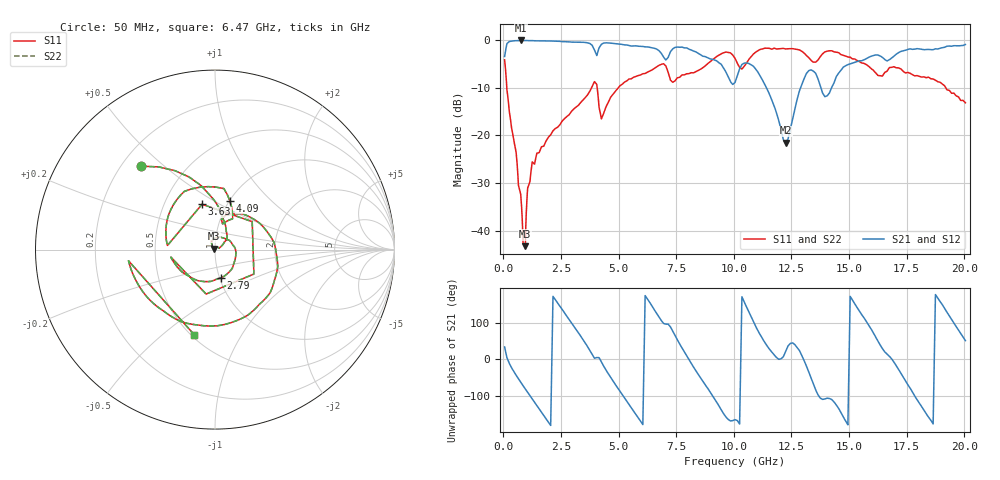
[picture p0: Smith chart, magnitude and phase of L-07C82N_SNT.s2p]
#	mhz	s	ma	r	50
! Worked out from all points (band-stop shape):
!   1001 points, 50 MHz to 20.05 GHz, reference 50 ohm
!   highest |S21| = -0.09 dB at 750 MHz (marker M1); lowest = -21.5 dB at 12.25 GHz (marker M2)
!   |S21| within 3 dB of the highest: 61.95 MHz to 4.037 GHz (3.975 GHz wide, 194 % of centre); 17.02 GHz to end of sweep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
!   lowest |S11| = -43.2 dB at 950 MHz (marker M3), VSWR 1.01, Z = 49.6 + j0.535 ohm
!   |S11| at or under -10 dB: 145.2 MHz to 3.826 GHz (3.681 GHz wide, 185 % of centre); 4.069 GHz to 4.986 GHz (917.5 MHz wide, 20.3 % of centre); 19.2 GHz to end of sweep
!   |S22| runs from -43.2 to -1.7 dB; largest |S21 - S12| = 0
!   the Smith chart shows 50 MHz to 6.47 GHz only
!   S11 on the Smith chart (normalised r, x): 50 MHz: 0.28, +0.42; 2.79 GHz: 1.01, -0.33; 3.63 GHz: 0.77, +0.42; 4.09 GHz: 1.00, +0.60; 6.47 GHz: 0.52, -0.65
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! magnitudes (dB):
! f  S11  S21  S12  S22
! 50 MHz  -4.1  -3.5  -3.5  -4.1
! 750 MHz  -32.4  -0.1  -0.1  -32.4
! 870 MHz  -42.7  -0.1  -0.1  -42.7
! 950 MHz  -43.2  -0.1  -0.1  -43.2
! 1.13 GHz  -29.9  -0.1  -0.1  -29.9
! 1.33 GHz  -25.9  -0.2  -0.2  -25.9
! 2.79 GHz  -15.9  -0.4  -0.4  -15.9
! 3.39 GHz  -12.9  -0.5  -0.5  -12.9
! 3.63 GHz  -11.6  -0.6  -0.6  -11.6
! 4.09 GHz  -10.9  -2.6  -2.6  -10.9
! 4.31 GHz  -15.8  -0.7  -0.7  -15.8
! 6.47 GHz  -6.2  -1.7  -1.7  -6.2
! 6.73 GHz  -5.4  -2.2  -2.2  -5.4
! 7.37 GHz  -8.8  -1.8  -1.8  -8.8
! 10.05 GHz  -3.8  -8.9  -8.9  -3.8
! 10.91 GHz  -2.7  -5.9  -5.9  -2.7
! 12.25 GHz  -1.9  -21.5  -21.5  -1.9
! 13.39 GHz  -4.4  -6.4  -6.4  -4.4
! 14.01 GHz  -2.4  -11.8  -11.8  -2.4
! 14.85 GHz  -3.4  -5.4  -5.4  -3.4
! 16.73 GHz  -5.9  -4.2  -4.2  -5.9
! 20.05 GHz  -13.2  -0.9  -0.9  -13.2
